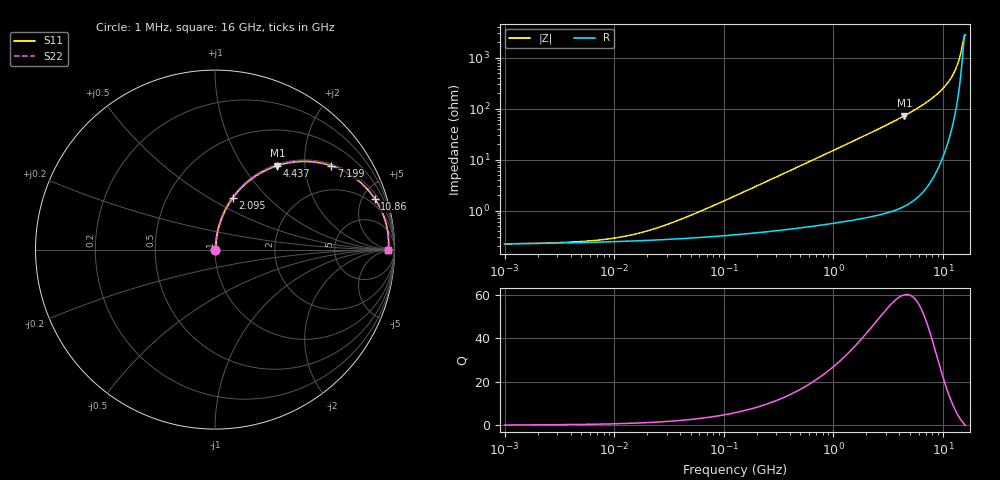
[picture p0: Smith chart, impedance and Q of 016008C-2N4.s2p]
# MHz S MA R 50
!Freq  MagS11  AngS11  MagS21  AngS21  MagS12  AngS12  MagS22  AngS22
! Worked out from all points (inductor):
!   801 points, 1 MHz to 16 GHz, reference 50 ohm
!   read as one part in series: L = 2.4 nH near 59.02 MHz
!   highest Q = 60.1 at 4.437 GHz (marker M1), where L = 2.6 nH
!   self-resonance near 15.9 GHz
!   S11 on the Smith chart (normalised r, x): 1 MHz: 1.00, +0.00; 2.095 GHz: 1.01, +0.64; 4.437 GHz: 1.02, +1.45; 7.199 GHz: 1.06, +2.73; 10.86 GHz: 1.37, +6.14; 16 GHz: 56, -8
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1  0.00221 3.9  0.9978 -0.0  0.9978 -0.0  0.00221 3.9
5.060461  0.002463 18.0  0.9977 -0.0  0.9977 -0.0  0.002463 18.0
11.80458  0.003044 35.6  0.9975 -0.1  0.9975 -0.1  0.003044 35.6
17.17751  0.00363 45.2  0.9974 -0.1  0.9974 -0.1  0.00363 45.2
25.30026  0.004635 55.0  0.9973 -0.2  0.9973 -0.2  0.004635 55.0
49.22189  0.007936 68.4  0.9971 -0.4  0.9971 -0.4  0.007936 68.4
128.031  0.01953 79.1  0.9965 -1.1  0.9965 -1.1  0.01953 79.1
317.2864  0.04779 82.4  0.9948 -2.7  0.9948 -2.7  0.04779 82.4
640.1033  0.09589 81.6  0.9906 -5.5  0.9906 -5.5  0.09589 81.6
1186.486  0.1762 78.0  0.9786 -10.1  0.9786 -10.1  0.1762 78.0
2095.341  0.3042 71.0  0.9457 -17.7  0.9457 -17.7  0.3042 71.0
3200.258  0.4462 62.5  0.8868 -26.5  0.8868 -26.5  0.4462 62.5
4436.843  0.5829 53.4  0.8029 -35.6  0.8029 -35.6  0.5829 53.4
5720.477  0.6981 44.7  0.704 -44.3  0.704 -44.3  0.6981 44.7
7199.131  0.799 35.8  0.5844 -53.0  0.5844 -53.0  0.799 35.8
9059.994  0.8849 25.9  0.4367 -62.2  0.4367 -62.2  0.8849 25.9
10863.14  0.9345 17.7  0.3038 -68.9  0.3038 -68.9  0.9345 17.7
12260.46  0.9559 12.1  0.21 -71.9  0.21 -71.9  0.9559 12.1
13344.21  0.9648 8.1  0.1434 -71.8  0.1434 -71.8  0.9648 8.1
14176.48  0.9679 5.3  0.09649 -67.9  0.09649 -67.9  0.9679 5.3
15429.6  0.9676 1.4  0.04015 -35.5  0.04015 -35.5  0.9676 1.4
16000  0.9659 -0.3  0.0345 8.1  0.0345 8.1  0.9659 -0.3
